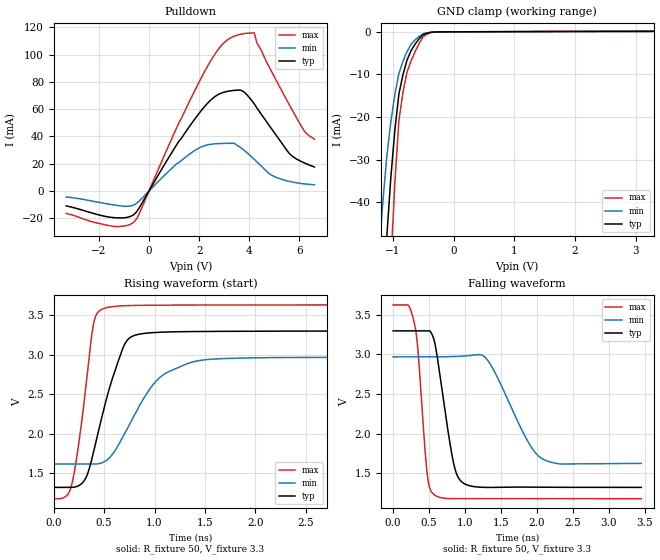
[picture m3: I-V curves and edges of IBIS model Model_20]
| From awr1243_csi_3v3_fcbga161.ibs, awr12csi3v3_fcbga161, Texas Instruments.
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| Model based on original model for BC1833DV40DCPBFBP18LL_OD_FS_SSDLV
|   Sub model BC40D_V_PD_ON_10P_!SC1_3P3
[model]   Model_20
|[Description]  [3.3V-I/O_OPEN_DRAIN-WEAK_PD_ON-FAST, IND, 10%]
|   FAST,WEAK_PD_ON,IND,10%
|[Input Load]   WEAK_PD_ON
|[Output Drive] FAST
|Voltage   3.3V
|Mode   I/O_OPEN_DRAIN
Model_type   I/O_open_drain
Polarity   Non-Inverting
Enable   Active-Low
Vinl =  0.8V
Vinh =  2V
Cref =  15pF
Rref =  100.0000M
Vref =  0V
Vmeas =  1.65
C_comp   2.059994p   1.912853p   2.135747p
[Model Spec]
Vinl   0.8V   0.8V   0.8V
Vinh   2V   2V   2V
[Temperature Range]   25   125   -40
[Voltage Range]   3.3   2.97   3.63
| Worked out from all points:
|   slope of the pulldown table from 0 to 0.495 V, typ, clamps not added: 31.8 ohm
|   GND clamp passes 1 mA (typ) near -0.52 V on its own axis
|   rising waveform, R_fixture 50, V_fixture 3.3: 20-80 % time 251ps typ, 385ps min, 142ps max; typ from 1.32 V to 3.3 V
|   falling waveform, R_fixture 50, V_fixture 3.3: 20-80 % time 196ps typ, 423ps min, 118ps max; typ from 3.3 V to 1.32 V
[Pulldown]
-3.3V     -10.92mA   -4.307mA   -16.45mA
-1.4V     -19.52mA   -10.22mA   -25.94mA
-600mV    -17.22mA   -10.25mA   -22.66mA
1.1V      33.8mA     19.88mA    46.22mA
2.1V      59.3mA     32.44mA    83.48mA
2.9V      71.86mA    34.84mA    107mA
3.5V      73.95mA    33.66mA    114.2mA
4.2V      63.8mA     23.19mA    116mA
4.9V      45.33mA    11.53mA    87.2mA
5.6V      27.47mA    7.046mA    63.1mA
6.2V      20.56mA    5.221mA    43.87mA
6.6V      17.6mA     4.555mA    38.05mA
[GND_clamp]
-3.3V     -787.2mA   -607.8mA   -1.235A
-1.233V   -85.66mA   -52.14mA   -138.8mA
-1.167V   -66.47mA   -40.37mA   -107.7mA
-1.1V     -48.25mA   -29.37mA   -77.99mA
-1.033V   -34.28mA   -21.19mA   -54.56mA
-966.7mV  -23.07mA   -14.67mA   -35.51mA
-900mV    -14.62mA   -9.792mA   -20.84mA
-833.3mV  -10.07mA   -6.938mA   -14.17mA
-700mV    -4.435mA   -2.939mA   -6.836mA
-500mV    -641.2uA   -454.5uA   -1.12mA
-300mV    -31.62uA   -32.73uA   -44.27uA
3.3V      108.6uA    159.4uA    198.5uA
[Ramp]
dV/dt_f  1.1955291/0.19759124n 0.83566775/0.43944611n  1.4751133/0.11837667n
dV/dt_r  1.1907008/0.23427848n 0.82841557/0.48868592n  1.4893273/0.136982n
R_load = 50
[Rising Waveform]
R_fixture = 50
V_fixture = 3.3
V_fixture_min = 2.97
V_fixture_max = 3.63
0s        1.321V     1.616V     1.179V
178.4ps   1.321V     1.616V     1.359V
304.7ps   1.412V     1.616V     2.443V
385.5ps   1.721V     1.616V     3.326V
470.7ps   2.176V     1.629V     3.567V
685.4ps   3.081V     1.957V     3.616V
810.9ps   3.246V     2.26V      3.62V
1.06ns    3.282V     2.718V     3.624V
1.411ns   3.291V     2.915V     3.625V
3.453ns   3.297V     2.965V     3.627V
[Falling Waveform]
R_fixture = 50
V_fixture = 3.3
V_fixture_min = 2.97
V_fixture_max = 3.63
0s        3.298V     2.97V      3.626V
295.6ps   3.298V     2.97V      3.395V
344ps     3.298V     2.97V      3.07V
474ps     3.298V     2.97V      1.491V
571.3ps   3.178V     2.97V      1.228V
832.9ps   1.662V     2.974V     1.179V
967ps     1.381V     2.979V     1.179V
1.312ns   1.32V      2.931V     1.179V
2.078ns   1.323V     1.682V     1.178V
3.453ns   1.321V     1.624V     1.178V
